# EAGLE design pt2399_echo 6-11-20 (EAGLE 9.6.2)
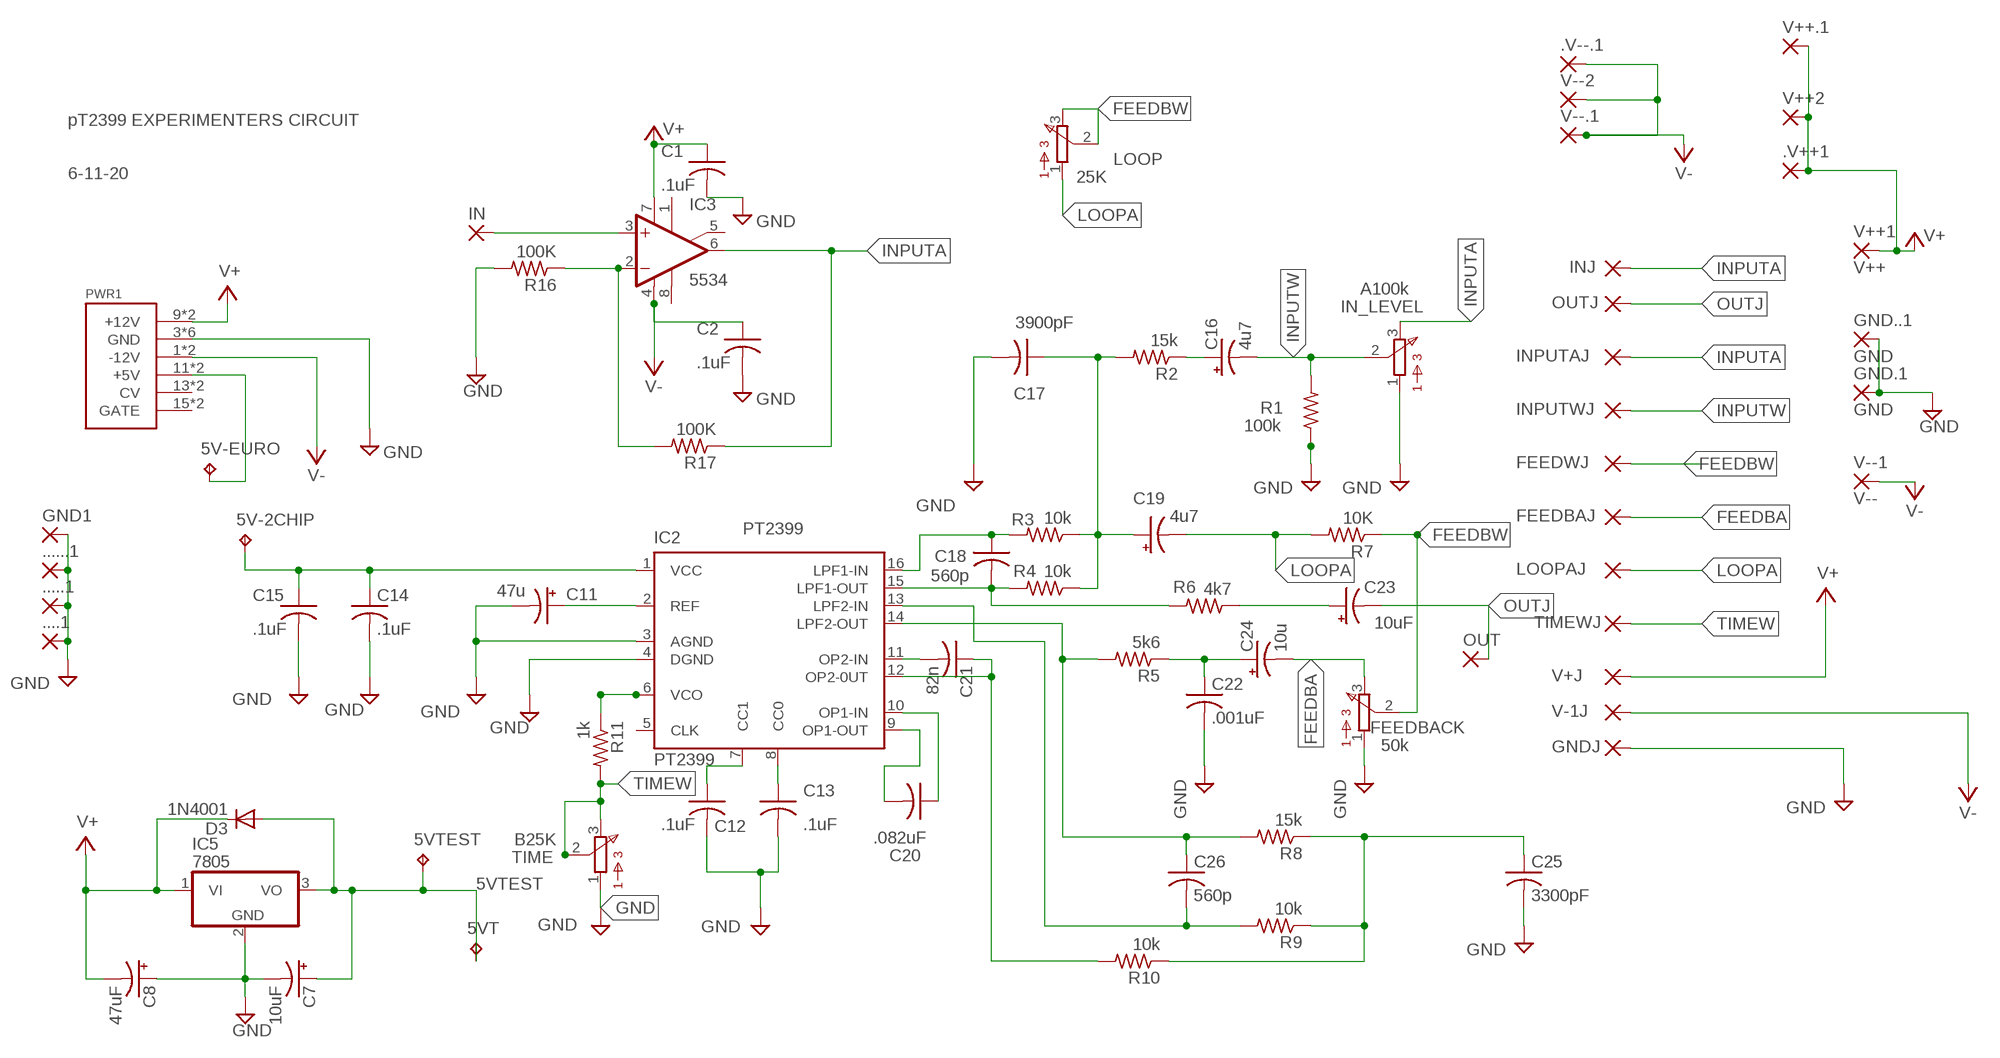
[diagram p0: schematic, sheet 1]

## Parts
5V-2CHIP  TPPAD1-13  [P1-13]
5V-EURO  TPPAD1-13  [P1-13]
5VT  TPPAD1-13  [P1-13]
5VTEST  TPPAD1-13  [P1-13]
....1  3,17/1,3  [3,17/1,3]
.....1  3,17/1,3  [3,17/1,3]
......1  3,17/1,3  [3,17/1,3]
.V++1  2,54/1,0  [2,54/1,0]
.V--.1  3,17/1,3  [3,17/1,3]
C1  .1uF  C-US025-030X050  [C025-030X050]
C2  .1uF  C-US025-030X050  [C025-030X050]
C7  10uF  CPOL-USTT5D7  [TT5D7]
C8  47uF  CPOL-USTT5D7  [TT5D7]
C11  47u  CPOL-USTT5D7  [TT5D7]
C12  .1uF  C-US025-030X050  [C025-030X050]
C13  .1uF  C-US025-030X050  [C025-030X050]
C14  .1uF  C-US025-030X050  [C025-030X050]
C15  .1uF  C-US025-030X050  [C025-030X050]
C16  4u7  CPOL-USTT5D7  [TT5D7]
C17  3900pF  C-US050-045X075  [C050-045X075]
C18  560p  C-US050-024X044  [C050-024X044]
C19  4u7  CPOL-USE5-5  [E5-5]
C20  .082uF  C-US050-025X075  [C050-025X075]
C21  82n  C-US050-025X075  [C050-025X075]
C22  .001uF  C-US025-040X050  [C025-040X050]
C23  10uF  CPOL-USTT2D7  [TT2D7]
C24  10u  CPOL-USTT5D7  [TT5D7]
C25  3300pF  C-US050-045X075  [C050-045X075]
C26  560p  C-US050-024X044  [C050-024X044]
D3  1N4001  1N4148DO35-10  [DO35-10]
FEEDBACK  50k  308/309  [308]
FEEDBAJ  WIREPAD1,6/0,9  [1,6/0,9]
FEEDWJ  WIREPAD1,6/0,9  [1,6/0,9]
GND1  3,17/1,3  [3,17/1,3]
GND.1  GND  1,6/0,8  [1,6/0,8]
GND..1  GND  1,6/0,8  [1,6/0,8]
GNDJ  WIREPAD1,6/0,9  [1,6/0,9]
IC2  PT2399  [DIP16]
IC3  5534  TL081P  [DIL08]
IC5  7805  7805T  [TO220H]
IN  3,17/1,3  [3,17/1,3]
IN_LEVEL  A100k  308/309  [308]
INJ  WIREPAD1,6/0,9  [1,6/0,9]
INPUTAJ  WIREPAD1,6/0,9  [1,6/0,9]
INPUTWJ  WIREPAD1,6/0,9  [1,6/0,9]
LOOP  25K  308/309  [308]
LOOPAJ  WIREPAD1,6/0,9  [1,6/0,9]
OUT  3,17/1,3  [3,17/1,3]
OUTJ  WIREPAD1,6/0,9  [1,6/0,9]
PWR1  POWER  [POWER_16]
R1  100k  R-US_0207/10  [0207/10]
R2  15k  R-US_0207/10  [0207/10]
R3  10k  R-US_0207/10  [0207/10]
R4  10k  R-US_0207/10  [0207/10]
R5  5k6  R-US_0207/10  [0207/10]
R6  4k7  R-US_0207/10  [0207/10]
R7  10K  R-US_0207/10  [0207/10]
R8  15k  R-US_0207/10  [0207/10]
R9  10k  R-US_0207/10  [0207/10]
R10  10k  R-US_0207/10  [0207/10]
R11  1k  R-US_0207/10  [0207/10]
R16  100K  R-US_0204/7  [0204/7]
R17  100K  R-US_0204/7  [0204/7]
TIME  B25K  308/309  [308]
TIMEWJ  WIREPAD1,6/0,9  [1,6/0,9]
V++1  V++  1,6/0,8  [1,6/0,8]
V++2  2,54/1,0  [2,54/1,0]
V++.1  2,54/1,0  [2,54/1,0]
V+J  WIREPAD1,6/0,9  [1,6/0,9]
V-1J  WIREPAD1,6/0,9  [1,6/0,9]
V--1  V--  1,6/0,8  [1,6/0,8]
V--2  3,17/1,3  [3,17/1,3]
V--.1  3,17/1,3  [3,17/1,3]

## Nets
5V+: 5V-2CHIP.TP C14.1 C15.1 IC2.1(VCC)
5VTEST: 5VT.TP 5VTEST.TP C7.+ D3.A IC5.3(VO)
FEEDBA: C24.- FEEDBACK.3 FEEDBAJ.1(P)
FEEDBW: FEEDBACK.2 FEEDWJ.1(P) LOOP.2 LOOP.3 R7.1
GND: ....1.1(P) .....1.1(P) ......1.1(P) C1.2 C2.2 C7.- C8.+ C11.- C12.2 C13.2 C14.2 C15.2 C17.2 C22.2 C25.2 FEEDBACK.1 GND1.1(P) GND.1.1(P) GND..1.1(P) GNDJ.1(P) IC2.3(AGND) IC2.4(DGND) IC5.2(GND) IN_LEVEL.1 PWR1.3(GND) PWR1.4(GND) PWR1.5(GND) PWR1.6(GND) PWR1.7(GND) PWR1.8(GND) R1.1 R16.2 TIME.1
INPUTA: IC3.6(OUT) IN_LEVEL.3 INJ.1(P) INPUTAJ.1(P) R17.1
INPUTW: C16.- IN_LEVEL.2 INPUTWJ.1(P) R1.2
LOOPA: C19.- LOOP.1 LOOPAJ.1(P) R7.2
N$1: IC3.3(+IN) IN.1(P)
N$2: 5V-EURO.TP PWR1.11(+5V) PWR1.12(+5V)
N$3: C23.+ R6.1
N$4: C12.1 IC2.7(CC1)
N$5: C13.1 IC2.8(CC0)
N$8: C11.+ IC2.2(REF)
N$9: C16.+ R2.1
N$11: C18.2 IC2.15(LPF1-OUT) R4.2 R6.2
N$12: C18.1 IC2.16(LPF1-IN) R3.2
N$13: C17.1 C19.+ R2.2 R3.1 R4.1
N$14: C20.2 IC2.9(OP1-OUT)
N$15: C20.1 IC2.10(OP1-IN)
N$16: C21.2 IC2.11(OP2-IN)
N$18: C26.1 IC2.14(LPF2-OUT) R5.2 R8.2
N$21: C22.1 C24.+ R5.1
N$23: C21.1 IC2.12(OP2-0UT) R10.2
N$24: C26.2 IC2.13(LPF2-IN) R9.2
N$25: C25.1 R8.1 R9.1 R10.1
N$28: IC3.2(-IN) R16.1 R17.2
N$29: IC2.6(VCO) R11.1
OUTJ: C23.- OUT.1(P) OUTJ.1(P)
TIMEW: R11.2 TIME.2 TIME.3 TIMEWJ.1(P)
V+: .V++1.1(P) C1.1 C8.- D3.C IC3.7(V+) IC5.1(VI) PWR1.9(+12V) PWR1.10(+12V) V++1.1(P) V++2.1(P) V++.1.1(P) V+J.1(P)
V-: .V--.1.1(P) C2.1 IC3.4(V-) PWR1.1(-12V) PWR1.2(-12V) V-1J.1(P) V--1.1(P) V--2.1(P) V--.1.1(P)
Unconnected: IC2.5(CLK) IC3.1(ON1) IC3.5(ON2) IC3.8(OPT) PWR1.13(CV) PWR1.14(CV) PWR1.15(GATE) PWR1.16(GATE)

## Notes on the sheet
- pT2399 EXPERIMENTERS CIRCUIT
- 6-11-20
- PT2399

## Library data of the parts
5V-2CHIP 5V-EURO 5VT 5VTEST = testpad:TP: Test pad
....1 .....1 ......1 GND1 IN OUT = wirepad:3,17/1,3: THROUGH-HOLE PAD
.V++1 V++2 V++.1 = wirepad-NONAMES:2,54/1,0: THROUGH-HOLE PAD
.V--.1 V--2 V--.1 = wirepad-NONAMES:3,17/1,3: THROUGH-HOLE PAD
C1 C2 C12-C15 C22 = rcl:C-US: CAPACITOR, American symbol; SPICEPREFIX: C
C7 C8 C11 C16 C23 C24 = resistor:CPOL-US: POLARIZED CAPACITOR, American symbol
C17 C25 = adafruit:C-US: CAPACITOR, American symbol
C18 C20 C21 C26 = rcl:C-US: CAPACITOR, American symbol
C19 = rcl:CPOL-US: POLARIZED CAPACITOR, American symbol; SPICEPREFIX: C
D3 = diode:1N4148: DIODE
FEEDBACK IN_LEVEL LOOP TIME = bourns:308/309: 308/309 Series Potentiometer
FEEDBAJ FEEDWJ GNDJ INJ INPUTAJ INPUTWJ LOOPAJ OUTJ TIMEWJ V+J V-1J = wirepad-NONAMES:WIREPAD: Wire PAD connect wire on PCB
GND.1 GND..1 V++1 V--1 = wirepad-NONAMES:1,6/0,8: THROUGH-HOLE PAD
IC2 = echounit:PT2399: Echo Processor IC
IC3 = linear:TL081: OP AMP
IC5 = linear:78*: Positive VOLTAGE REGULATOR Source: http://cache.national.com/ds/LM/LM78L05.pdf http://www.fairchildsemi.com/ds/LM/LM7805.pdf
PWR1 = eurorack:POWER
R1-R11 = resistor:R-US_: RESISTOR, American symbol
R16 R17 = rcl:R-US_: RESISTOR, American symbol

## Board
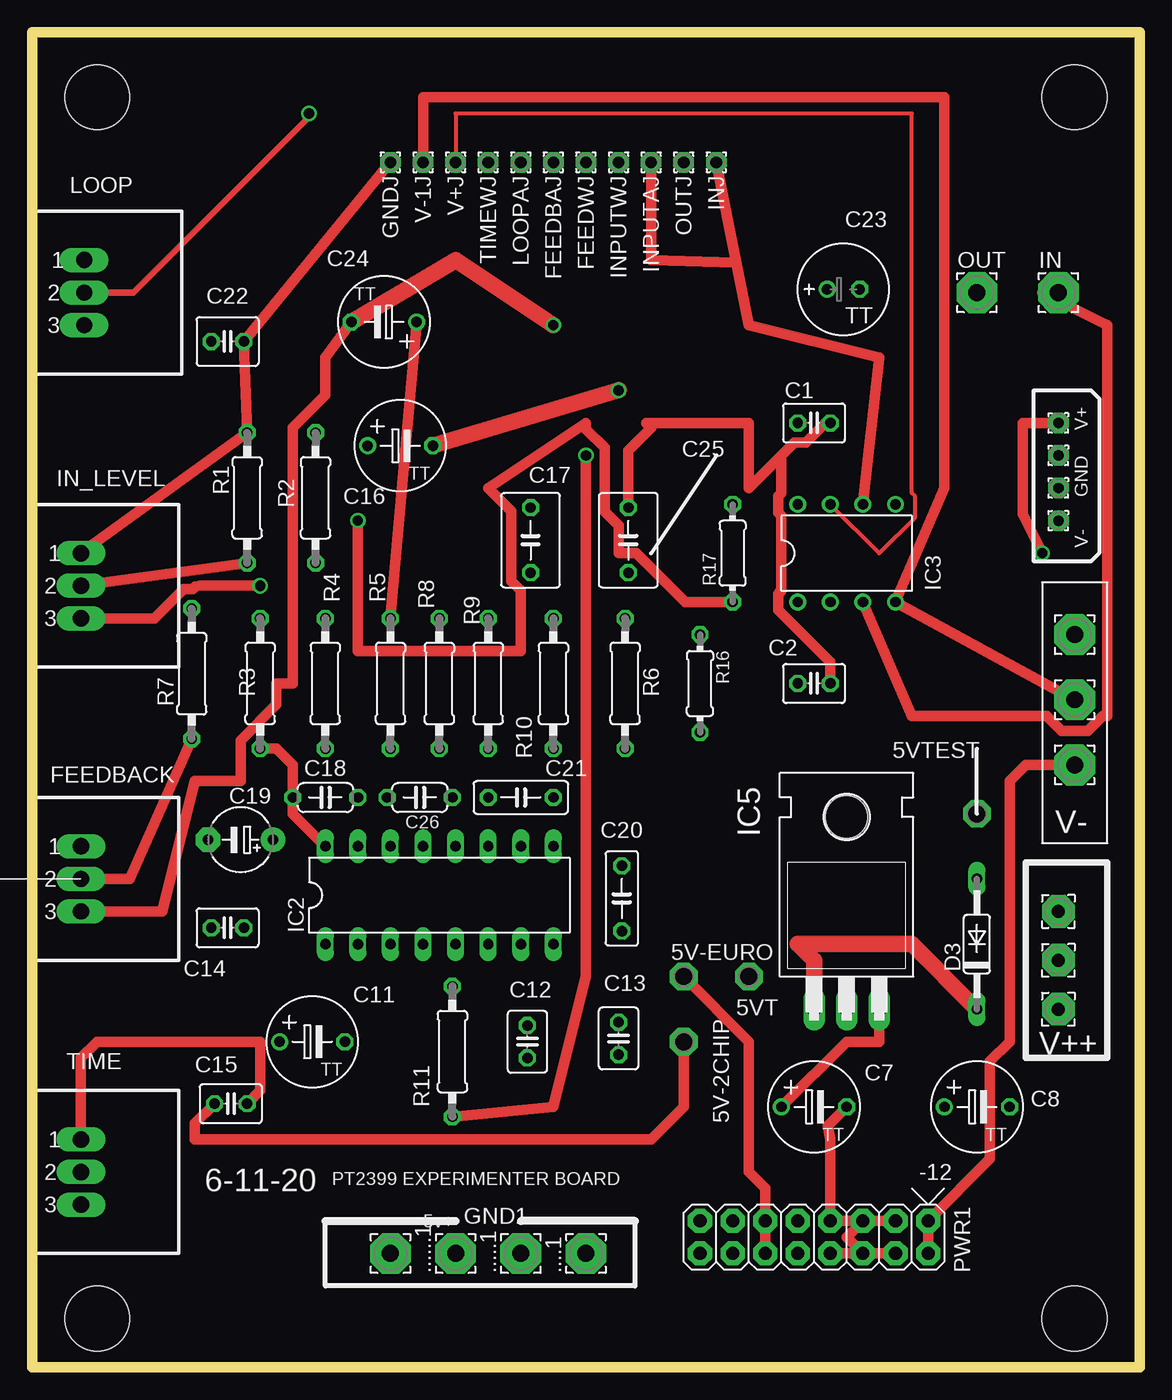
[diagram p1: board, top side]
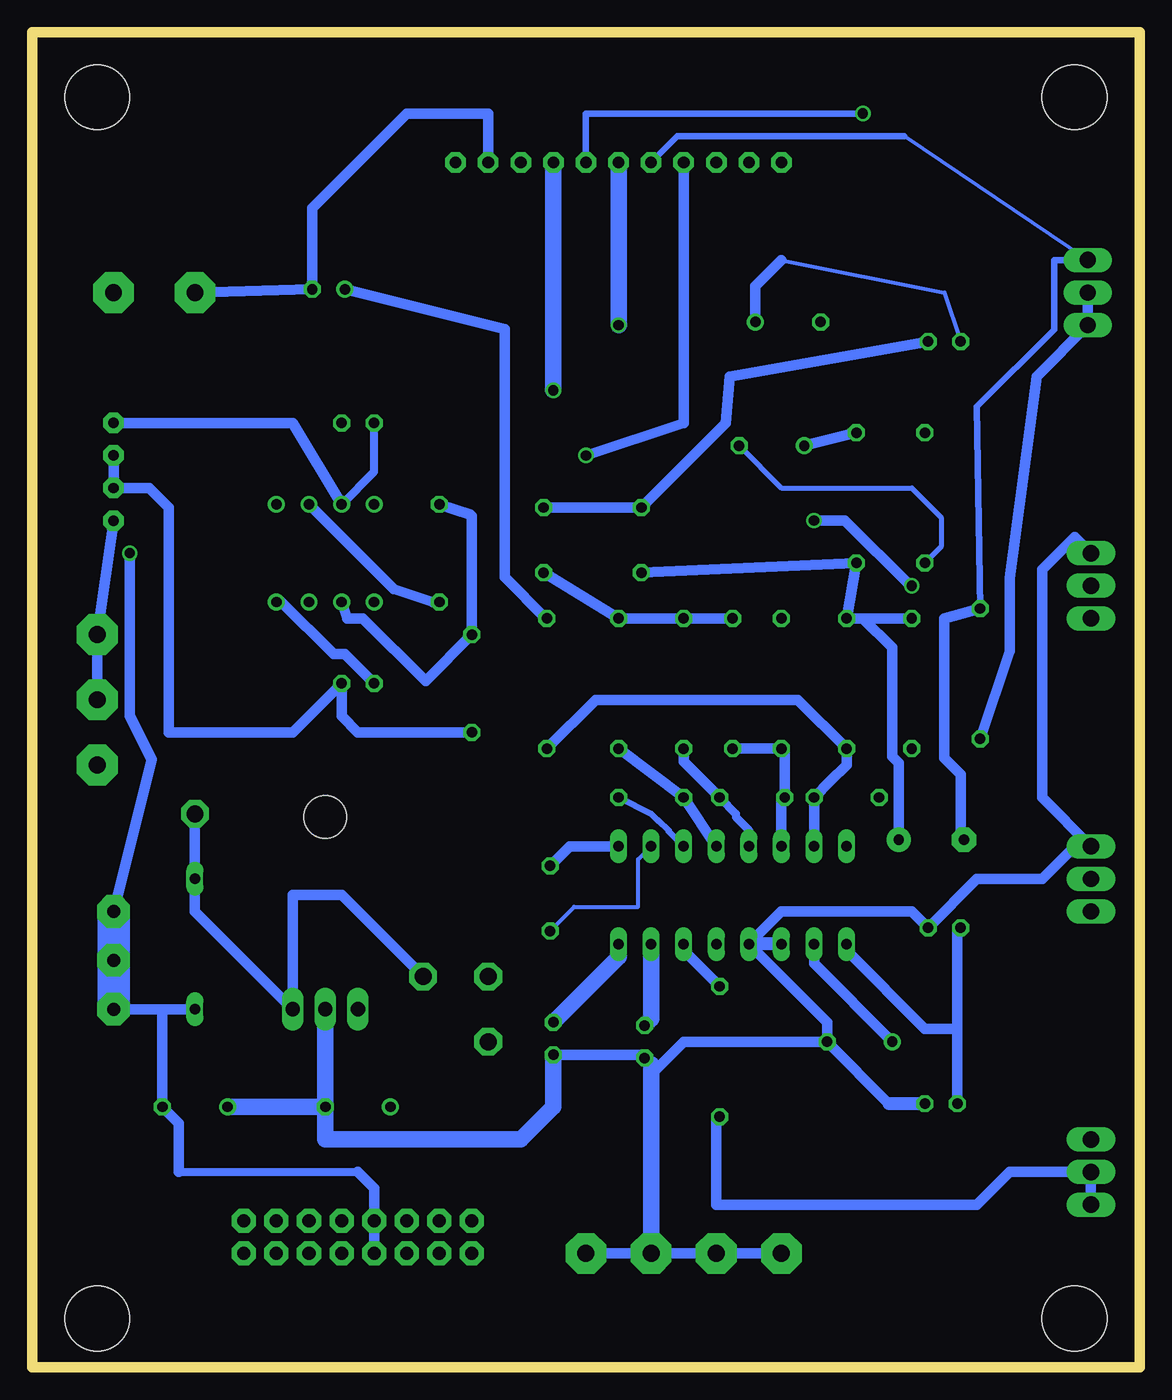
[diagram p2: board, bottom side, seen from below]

Size 86.36 x 104.14 mm. Coordinates in mm from the lower left corner, seen from the top.
Outline: 0,104.14 0,0 86.36,0 86.36,104.14 0,104.14
Copper layers (1*16): Top 0.035mm / dielectric 1.5mm / Bottom 0.035mm
Design rules "default *": minimum track width 12mil, minimum drill 31mil, track to track 18mil, track to pad 18mil, pad to pad 18mil, via to via 18mil, smd to smd 8mil, copper to edge 0mil, drill to drill 18mil, minimum pad ring 10mil, minimum via ring 8mil, stop-mask expansion 4mil, vias tented up to drill 0mil, thermal gap 10mil
Holes 5.08 mm at 5.08,99.06 81.28,99.06 81.28,3.81 5.08,3.81

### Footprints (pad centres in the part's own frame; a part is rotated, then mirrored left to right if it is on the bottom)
P1-13 = drill 1.321 pad 2.159 octagon: TP 0,0
3,17/1,3 = drill 1.321 pad 3.175 octagon: 1 0,0
2,54/1,0 = drill 1.016 pad 2.54 octagon: 1 0,0
C025-030X050 = drill 0.813 octagon: 1 -1.27,0; 2 1.27,0
TT5D7 = drill 0.813: + -2.54,0 | drill 0.813 octagon: - 2.54,0
C050-045X075 = drill 0.813 octagon: 1 -2.54,0; 2 2.54,0
C050-024X044 = drill 0.813 octagon: 1 -2.54,0; 2 2.54,0
E5-5 = drill 0.813 pad 1.905: + -2.54,0 | drill 0.813 pad 1.905 octagon: - 2.54,0
C050-025X075 = drill 0.813 octagon: 1 -2.54,0; 2 2.54,0
C025-040X050 = drill 0.813 octagon: 1 -1.27,0; 2 1.27,0
TT2D7 = drill 0.813: + -1.27,0 | drill 0.813 octagon: - 1.27,0
DO35-10 = drill 0.813 long: A 5.08,0; C -5.08,0
308 = drill 1.27 long: 1 0,2.54; 2 0,0; 3 0,-2.54
1,6/0,9 = drill 0.914 pad 1.6 octagon: 1 0,0
1,6/0,8 = drill 0.813 pad 1.6 octagon: 1 0,0
DIP16 = drill 0.813 long: 1 -7.62,-3.81; 2 -5.08,-3.81; 3 -2.54,-3.81; 4 0,-3.81; 5 2.54,-3.81; 6 5.08,-3.81; 7 7.62,-3.81; 8 10.16,-3.81; 9 10.16,3.81; 10 7.62,3.81; 11 5.08,3.81; 12 2.54,3.81; 13 0,3.81; 14 -2.54,3.81; 15 -5.08,3.81; 16 -7.62,3.81
DIL08 = drill 0.813 pad 1.27: 1 -3.81,-3.81; 2 -1.27,-3.81; 3 1.27,-3.81; 4 3.81,-3.81; 5 3.81,3.81; 6 1.27,3.81; 7 -1.27,3.81; 8 -3.81,3.81
TO220H = drill 1.118 long: 1 -2.54,-10.16; 2 0,-10.16; 3 2.54,-10.16 | hole 3.302: 0,4.826
POWER_16 = drill 1.016 pad 1.88 octagon: 1 -6.35,-1.27; 2 -6.35,1.27; 3 -3.81,-1.27; 4 -3.81,1.27; 5 -1.27,-1.27; 6 -1.27,1.27; 7 1.27,-1.27; 8 1.27,1.27; 9 3.81,-1.27; 10 3.81,1.27; 11 6.35,-1.27; 12 6.35,1.27; 13 8.89,-1.27; 14 8.89,1.27; 15 11.43,-1.27; 16 11.43,1.27
0207/10 = drill 0.813 octagon: 1 -5.08,0; 2 5.08,0
0204/7 = drill 0.813 octagon: 1 -3.81,0; 2 3.81,0

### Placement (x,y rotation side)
5V-2CHIP  50.8,25.4 0 top
5V-EURO  50.8,30.48 0 top
5VT  55.88,30.48 0 top
5VTEST  73.66,43.18 0 top
....1  43.18,8.89 90 top
.....1  38.1,8.89 90 top
......1  33.02,8.89 90 top
.V++1  80.01,31.75 0 top
.V--.1  81.28,46.99 0 top
C1  60.96,73.66 0 top
C2  60.96,53.34 0 top
C7  60.96,20.32 0 top
C8  73.66,20.32 0 top
C11  21.84,25.4 0 top
C12  38.61,25.4 270 top
C13  45.72,25.65 270 top
C14  15.24,34.29 0 top
C15  15.49,20.57 0 top
C16  28.7,71.88 0 top
C17  38.86,64.52 90 top
C18  22.86,44.45 0 top
C19  16.26,41.15 180 top
C20  45.97,36.58 90 top
C21  38.1,44.45 0 top
C22  15.24,80.01 0 top
C23  63.25,84.07 0 top
C24  27.43,81.53 180 top
C25  46.48,64.52 90 top
C26  30.23,44.45 0 top
D3  73.66,33.02 90 top
FEEDBACK  3.81,38.1 0 top
FEEDBAJ  40.64,93.98 270 top
FEEDWJ  43.18,93.98 270 top
GND1  27.94,8.89 90 top
GND.1  80.01,68.58 270 top
GND..1  80.01,71.12 270 top
GNDJ  27.94,93.98 270 top
IC2  30.48,36.83 0 top
IC3  63.5,63.5 0 top
IC5  63.5,38.1 0 top
IN  80.01,83.82 0 top
IN_LEVEL  3.81,60.96 0 top
INJ  53.34,93.98 270 top
INPUTAJ  48.26,93.98 270 top
INPUTWJ  45.72,93.98 270 top
LOOP  4.06,83.82 0 top
LOOPAJ  38.1,93.98 270 top
OUT  73.66,83.82 0 top
OUTJ  50.8,93.98 270 top
PWR1  63.5,10.16 180 top
R1  16.76,67.82 270 top
R2  22.1,67.82 270 top
R3  17.78,53.34 270 top
R4  22.86,53.34 270 top
R5  27.94,53.34 270 top
R6  46.23,53.34 270 top
R7  12.45,54.1 90 top
R8  31.75,53.34 270 top
R9  35.56,53.34 270 top
R10  40.64,53.34 270 top
R11  32.77,24.64 270 top
R16  52.07,53.34 270 top
R17  54.61,63.5 90 top
TIME  3.81,15.24 0 top
TIMEWJ  35.56,93.98 270 top
V++1  80.01,73.66 270 top
V++2  80.01,35.56 0 top
V++.1  80.01,27.94 0 top
V+J  33.02,93.98 270 top
V-1J  30.48,93.98 270 top
V--1  80.01,66.04 270 top
V--2  81.28,52.07 0 top
V--.1  81.28,57.15 0 top

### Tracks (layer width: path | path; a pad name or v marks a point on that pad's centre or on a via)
5V+
  Top 0.813: 5V-2CHIP.TP 50.8,20.32 48.26,17.78 12.7,17.78 12.7,19.05 C15.1
  Bottom 0.813: C15.1 14.22,26.42 | 14.22,26.42 14.22,34.04 C14.1 | IC2.1 22.86,32.51 16.76,26.42 14.22,26.42
5VTEST
  Top 0.813: C7.+ 63.5,25.4 66.04,25.4 IC5.3
  Bottom 0.813: 5VTEST.TP D3.A 73.66,35.56 IC5.3 66.04,36.83 62.23,36.83 5VT.TP
FEEDBA  (via drill 0.79)
  Top 0.813: FEEDBACK.3 10.16,35.56 12.7,45.72 16.26,45.72 16.26,48.89 19.05,51.69 19.05,53.34 20.32,53.34 20.32,73.28 22.86,75.81 22.86,78.74 C24.-
  Top 1.27: C24.- 33.02,86.36 v40.64,81.28
  Bottom 1.27: FEEDBAJ.1 v40.64,81.28
FEEDBW  (via drill 0.79)
  Top 0.508: LOOP.2 7.87,83.82 21.59,97.54 v21.59,97.79
  Top 0.813: R7.1 7.62,38.1 FEEDBACK.2
  Bottom 0.508: FEEDWJ.1 43.18,97.79 v21.59,97.79
  Bottom 0.813: R7.1 10.16,55.88 10.16,61.58 8.05,77.27 LOOP.3 LOOP.2
GND
  Top 0.813: PWR1.6 63.5,10.16 PWR1.5 PWR1.3 PWR1.7 62.23,17.81 62.02,18.84 C7.- | PWR1.4 PWR1.6 | C15.2 17.78,21.59 17.78,25.4 5.08,25.4 3.81,24.13 TIME.1 | IN_LEVEL.1 R1.1 C22.2 GNDJ.1 | C2.2 62.23,54.99 58.17,59.06 58.17,60.32 58.42,60.58 58.42,66.42 58.17,66.68 58.17,67.94 58.42,68.19 58.42,71.12 | 58.42,71.12 55.88,68.58 55.88,73.66 47.88,73.66 48.26,73.28 46.48,71.5 C25.2 | 58.42,71.12 59.44,72.14 60.32,72.14 61.84,73.66 C1.2 | PWR1.6 PWR1.8
  Bottom 0.813: ....1.1 .....1.1 ......1.1 GND1.1 | 38.1,23.62 C12.2 38.86,24.38 C13.2 | 63.5,17.78 C7.- | GND..1.1 GND.1.1 77.22,68.58 75.69,67.06 75.69,49.53 66.04,49.53 C2.2 62.23,50.8 60.96,49.53 R16.2 | C25.2 C17.2 32.28,73.64 31.98,77.28 C22.2 | IN_LEVEL.1 5.08,64.77 7.62,62.23 7.62,44.45 FEEDBACK.1 5.08,40.64 7.62,38.1 12.7,38.1 C14.2 17.78,35.56 27.94,35.56 IC2.4 24.38,26.92 C11.- | 38.1,22.86 35.56,25.4 C11.- | 19.56,20.57 C11.-
  Bottom 1.016: C15.2 19.56,20.57 | IC2.3 IC2.4
  Bottom 1.27: .....1.1 38.1,22.86 38.1,23.62 | C13.2 45.72,20.32 48.26,17.78 63.5,17.78 IC5.2 | C7.- C8.+
INPUTA  (via drill 0.79)
  Top 0.813: IC3.6 66.04,78.74 55.88,81.28 54.9,86.17 | 54.9,86.17 INJ.1 | 54.9,86.17 48.26,86.36 INPUTAJ.1 | v25.4,66.04 25.4,55.88 38.1,55.88 38.1,60.58 37.34,61.34 37.34,66.8 35.56,68.58 43.18,73.66 43.18,73.19 44.64,71.72 44.64,66.74 45.72,65.66 45.72,63.5 47.11,63.5 50.92,59.69 R17.1 | v17.78,60.96 13.15,60.96 12.71,60.9 12.52,60.71 11.81,60.71 9.53,58.42 IN_LEVEL.3
  Bottom 0.813: R17.1 55.12,59.69 58.17,60.71 IC3.6 | v25.4,66.04 22.99,66.04 17.91,60.96 v17.78,60.96
INPUTW  (via drill 0.79)
  Top 0.813: IN_LEVEL.2 R1.2
  Top 1.27: C16.- v45.72,76.2
  Bottom 0.406: C16.- 27.94,68.58 17.78,68.58 15.49,66.29 15.49,64.01 R1.2
  Bottom 1.27: INPUTWJ.1 v45.72,76.2
LOOPA
  Bottom 0.305: LOOP.1 18.35,96.01
  Bottom 0.508: LOOPAJ.1 36.07,96.01 18.35,96.01 | R7.2 12.7,74.93 6.68,80.95 6.68,86.36 LOOP.1
  Bottom 0.813: C19.- 13.97,41.4 13.97,46.25 15.24,47.52 15.24,58.42 R7.2
N$1
  Top 0.813: IC3.3 68.58,50.8 79.08,50.8 80.27,49.62 82.3,49.62 83.48,50.8 83.82,50.8 83.82,81.28 78.74,83.82 IN.1
N$2
  Top 0.813: 5V-EURO.TP 55.88,25.4 55.88,15.24 57.15,13.97 PWR1.11 PWR1.12
N$3
  Bottom 0.813: R6.1 46.32,58.42 49.53,61.63 49.53,80.96 C23.+
N$4
  Bottom 1.27: C12.1 38.1,27.18 IC2.7
N$5
  Bottom 0.813: 40.64,32 IC2.8
  Bottom 1.27: C13.1 40.64,32
N$8
  Bottom 0.813: C11.+ 25.4,31.5 IC2.2
N$9
  Bottom 0.813: R2.1 C16.+
N$11
  Bottom 0.813: R6.2 42.42,52.07 26.67,52.07 R4.2 22.86,46.99 24.13,45.72 C18.2 IC2.15
N$12
  Top 0.813: IC2.16 20.32,43.18 C18.1 20.32,46.99 19.05,48.26 R3.2
N$13
  Bottom 0.813: C17.1 R2.2 R4.1 21.59,58.42 | 21.59,58.42 R3.1 | C19.+ 18.8,47.12 19.3,47.63 19.3,56.13 21.59,58.42
N$14
  Bottom 0.813: C20.2 44.45,40.64 IC2.9
N$15
  Bottom 0.305: IC2.10 39.12,39.62 39.12,35.92 44.09,35.92 C20.1
N$16
  Bottom 0.508: IC2.11 36.73,41.81 36.73,41.87 37.53,42.67 37.59,42.67 38.1,43.18 C21.2
N$18
  Bottom 0.813: IC2.14 27.94,44.2 C26.1 27.69,48.01 R5.2 R8.2
N$21
  Top 0.813: C24.+ R5.1
  Bottom 0.305: 27.94,86.36 15.24,83.82 C22.1
  Bottom 0.813: C24.+ 29.97,84.33 27.94,86.36
N$23
  Bottom 0.813: IC2.12 C21.1 R10.2
N$24
  Bottom 0.61: C26.2 31.5,43.18 31.5,42.93 30.48,41.91 IC2.13
  Bottom 0.813: C26.2 35.56,47.24 R9.2
N$25
  Bottom 0.813: C25.1 R10.1 R9.1 R8.1
N$28
  Bottom 0.813: IC3.2 61.81,58.42 60.58,58.42 55.69,53.53 R16.1 52.07,66.39 52.19,66.5 R17.2
N$29
  Bottom 0.813: R11.1 35.56,32.51 IC2.6
OUTJ
  Bottom 0.813: OUT.1 C23.- 64.52,90.42 57.15,97.79 50.8,97.79 OUTJ.1
TIMEW  (via drill 0.79)
  Top 0.813: R11.2 40.64,20.32 43.18,30.48 v43.18,71.12
  Bottom 0.813: TIME.3 TIME.2 10.16,15.24 12.7,12.7 33.02,12.7 33.02,19.3 R11.2 | TIMEWJ.1 35.56,73.66 v43.18,71.12
V+  (via drill 0.79)
  Top 0.305: IC3.7 66.04,63.5 68.83,66.29 68.83,67.94 68.58,68.19 68.58,97.79 33.02,97.79 V+J.1
  Top 0.813: v78.74,63.5 77.22,66.55 77.22,73.66 V++1.1
  Top 1.27: IC5.1 60.96,31.75 59.69,33.02 68.58,33.02 D3.C
  Bottom 0.61: 74.93,15.24 60.96,15.24 | IC3.7 59.69,69.85 C1.1
  Bottom 0.813: V++.1.1 76.2,27.94 | 76.2,27.94 D3.C | 76.2,27.94 C8.- 74.93,19.05 74.93,15.24 | IC3.7 66.04,73.66 V++1.1 | V++2.1 77.05,47.41 78.74,50.8 v78.74,63.5 | PWR1.10 PWR1.9 59.69,13.97 60.96,15.24
  Bottom 2.54: V++2.1 .V++1.1 V++.1.1
V-
  Top 0.813: .V--.1.1 77.47,46.99 76.2,45.72 76.2,25.4 74.68,23.88 74.68,16.26 PWR1.1 PWR1.2 | V--2.1 IC3.4 71.12,68.58 71.12,99.06 30.48,99.06 V-1J.1
  Bottom 0.813: V--2.1 V--.1.1 V--1.1 | C2.1 61.98,55.63 62.86,55.63 66.92,59.69 IC3.4

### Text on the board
tNames: V+ | GND | V- | V- | V++ | 6-11-20 | PT2399 EXPERIMENTER BOARD | 5v+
